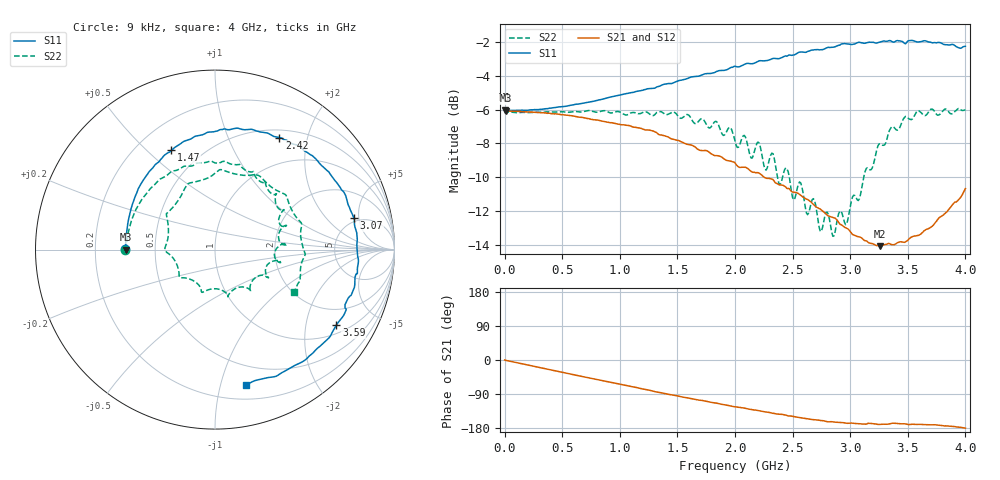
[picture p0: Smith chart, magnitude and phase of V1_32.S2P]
! ZVRE, 3.40
! symbol freq-unit parameter-type data-format keyword impedance-ohm
#  HZ  S  RI  R  50
! freq  reS11  imS11  reS21  imS21  reS12  imS12  reS22  imS22
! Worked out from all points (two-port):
!   401 points, 9 kHz to 4 GHz, reference 50 ohm
!   highest |S21| = -5.99 dB at 9 kHz (marker M1); lowest = -14.1 dB at 3.26 GHz (marker M2)
!   |S21| within 3 dB of the highest: start of sweep to 1.922 GHz
!   lowest |S11| = -6.1 dB at 10.01 MHz (marker M3), VSWR 2.98, Z = 16.8 + j0.00605 ohm
!   |S11| at or under -10 dB: nowhere
!   |S22| runs from -13.5 to -5.9 dB; largest |S21 - S12| = 0.0089
!   S11 on the Smith chart (normalised r, x): 9 kHz: 0.33, +0.00; 1.47 GHz: 0.34, +0.60; 2.42 GHz: 0.60, +1.56; 3.07 GHz: 4.54, +4.30; 3.59 GHz: 1.30, -2.98; 4 GHz: 0.32, -1.20
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9000  -0.4999 0.00141  0.5018 0.000846  0.5026 -0.00148  -0.5007 -0.000769
1.000898e7  -0.4978 0.000136  0.4962 -0.00773  0.4985 -0.00266  -0.4931 0.00865
6.700075e8  -0.4625 0.2449  0.3466 -0.3262  0.3522 -0.324  -0.3363 0.3616
1.340006e9  -0.2971 0.5076  0.0336 -0.4216  0.0361 -0.4256  0.0483 0.492
1.470006e9  -0.2427 0.5528  -0.0225 -0.4083  -0.019 -0.4104  0.1389 0.4732
1.820005e9  -0.0606 0.6431  -0.1432 -0.3377  -0.1428 -0.3397  0.341 0.3091
2.000004e9  0.0564 0.6722  -0.1927 -0.2904  -0.1906 -0.2909  0.36 0.1858
2.200004e9  0.1956 0.6699  -0.2244 -0.2366  -0.2221 -0.238  0.401 0.0283
2.260004e9  0.2365 0.6597  -0.2297 -0.2154  -0.227 -0.2172  0.3337 -0.0103
2.320004e9  0.2829 0.6511  -0.2391 -0.2005  -0.236 -0.2038  0.3654 -0.0726
2.420004e9  0.359 0.6242  -0.2419 -0.1755  -0.2413 -0.1766  0.289 -0.1471
2.670003e9  0.5449 0.5211  -0.2437 -0.1029  -0.2427 -0.1082  0.0726 -0.2612
2.850003e9  0.6537 0.4042  -0.2297 -0.0689  -0.2286 -0.0757  -0.1057 -0.1826
2.930002e9  0.7197 0.3177  -0.2196 -0.0592  -0.2218 -0.0579  -0.1997 -0.1447
3.070002e9  0.7749 0.1748  -0.2059 -0.0439  -0.2084 -0.0443  -0.2629 0.0591
3.150002e9  0.7864 0.1041  -0.1987 -0.0433  -0.1995 -0.0443  -0.2709 0.2005
3.260002e9  0.7952 -0.0396  -0.1942 -0.0346  -0.1954 -0.041  -0.1412 0.3712
3.340001e9  0.7933 -0.1323  -0.1969 -0.0392  -0.1978 -0.0407  0.012 0.4345
3.480001e9  0.7244 -0.3066  -0.1994 -0.0389  -0.2015 -0.0394  0.2411 0.4138
3.590001e9  0.6761 -0.4208  -0.209 -0.0372  -0.2126 -0.0397  0.3953 0.3036
3.82e9  0.427 -0.6555  -0.2449 -0.0257  -0.2467 -0.0272  0.5028 -0.024
4e9  0.171 -0.7541  -0.2923 -0.0013  -0.2915 0.000727  0.4411 -0.2378
